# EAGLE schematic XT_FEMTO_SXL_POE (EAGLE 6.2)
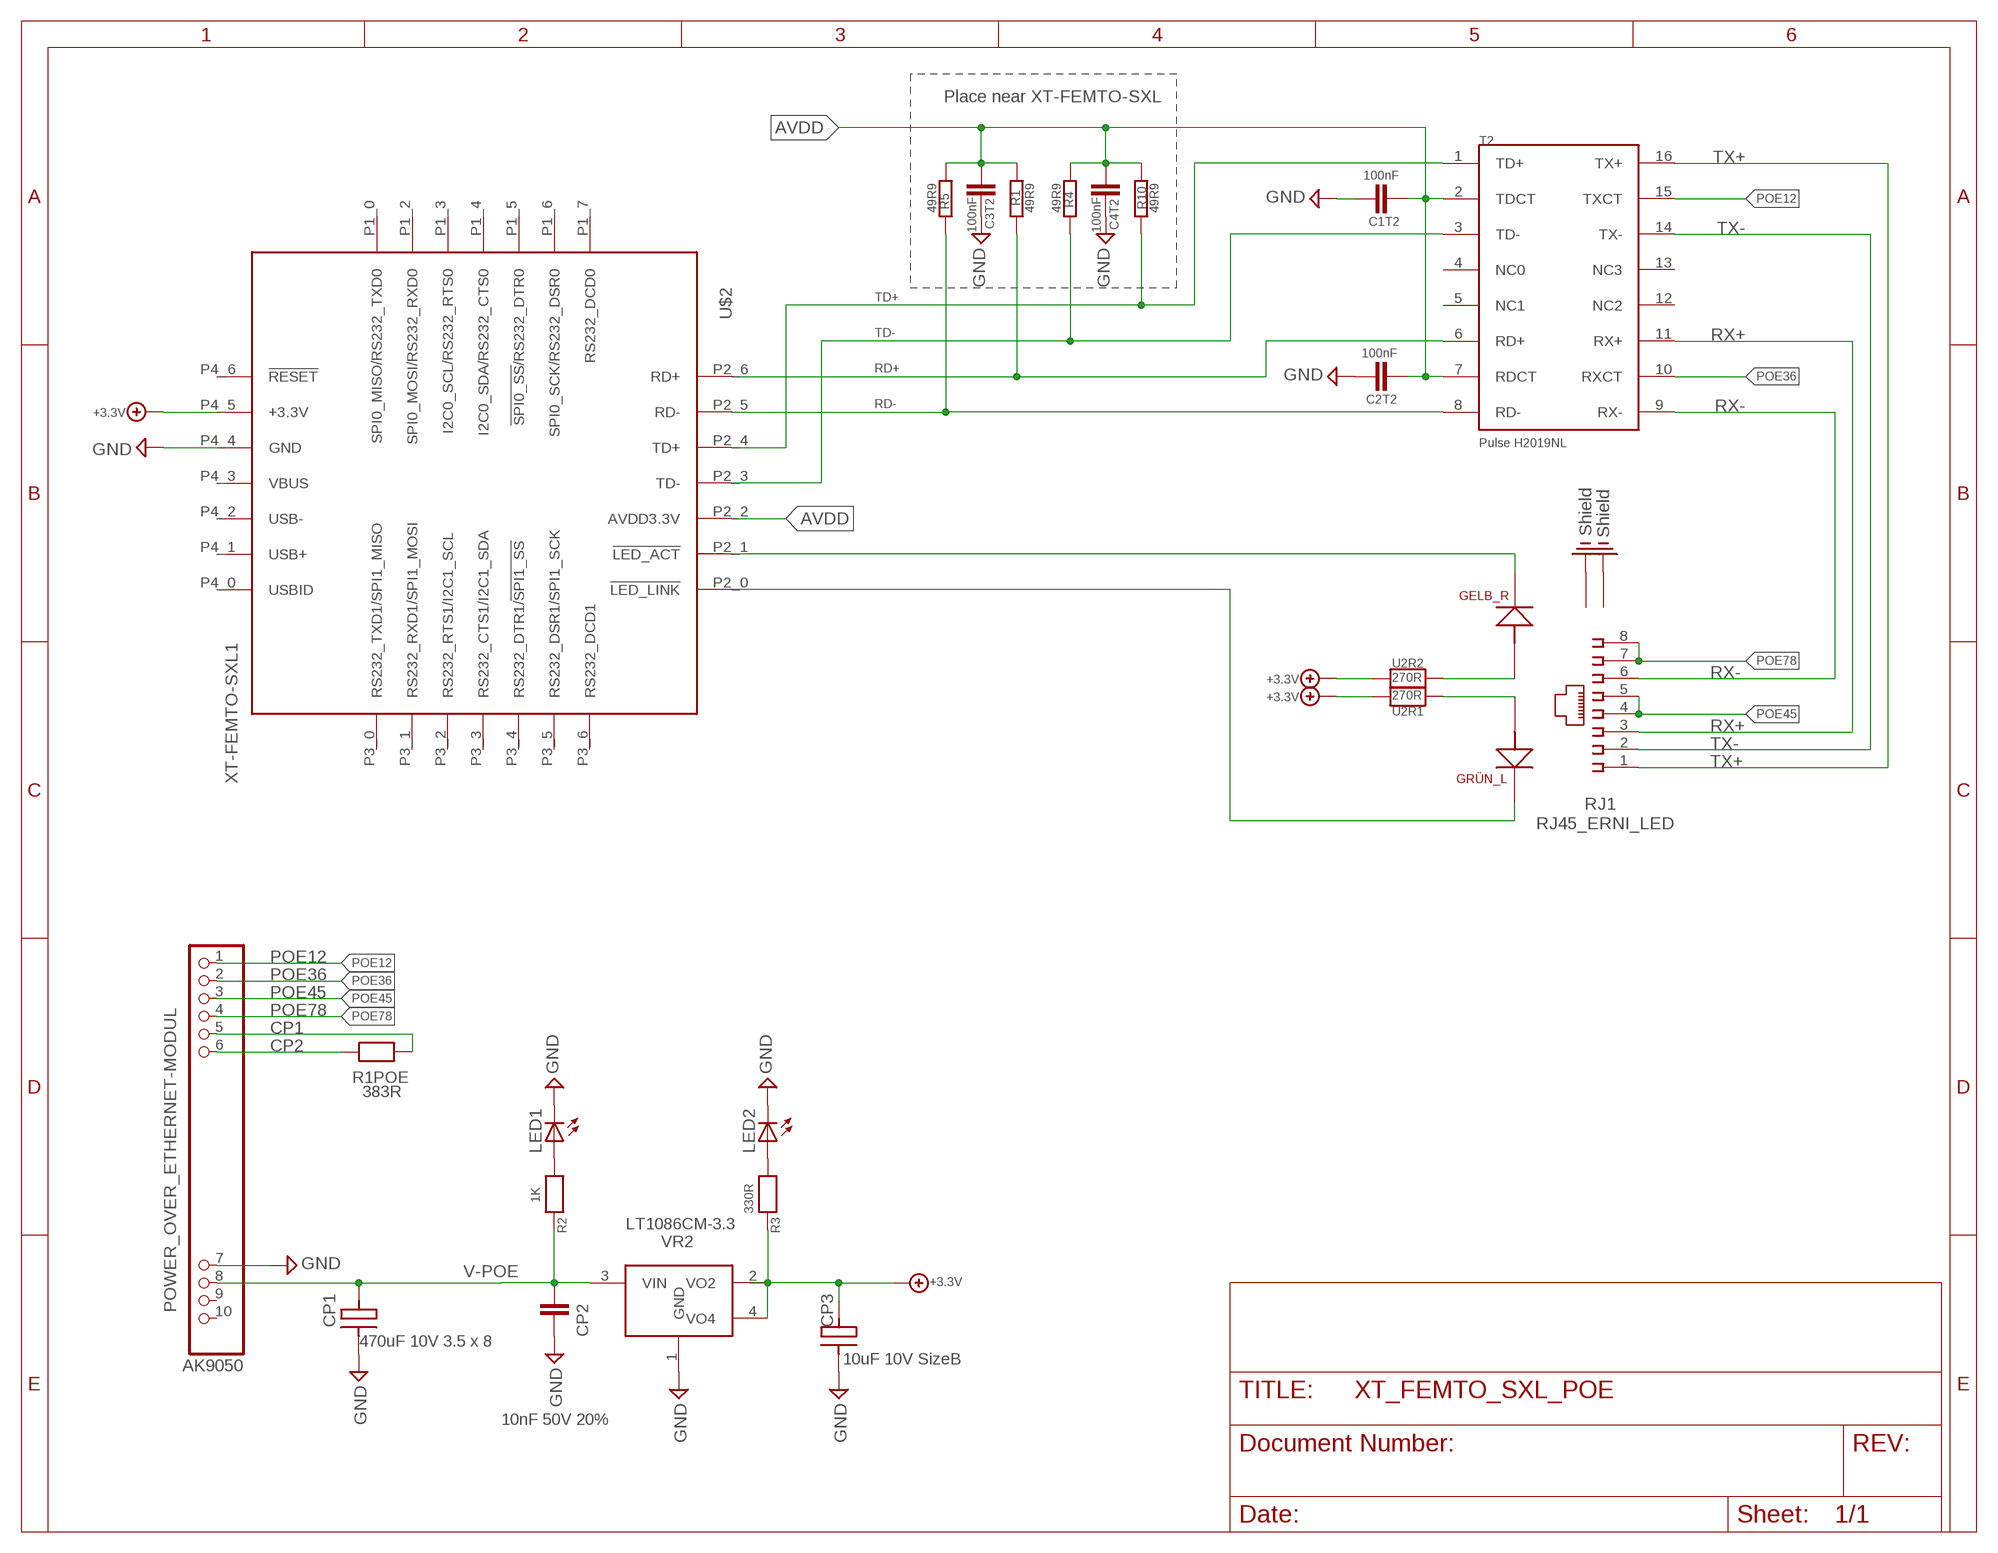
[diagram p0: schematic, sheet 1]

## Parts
C1T2  100nF  CHIP-C-VTS0402  [R0402_VTS]
C2T2  100nF  CHIP-C-VTS0402  [R0402_VTS]
C3T2  100nF  CHIP-C-VTS0402  [R0402_VTS]
C4T2  100nF  CHIP-C-VTS0402  [R0402_VTS]
CP1  470uF 10V 3.5 x 8  C3528_B  [ORCAD_X_CT3528]
CP2  10nF 50V 20%  CHIP-C-0603  [SMD-0603]
CP3  10uF 10V SizeB  C3528_B  [ORCAD_X_CT3528]
LED1  LED3MM  [LED3MM]
LED2  LED3MM  [LED3MM]
POWER_OVER_ETHERNET-MODUL  AK9050  POE_AG9000  [POE_AG9000]
R1  49R9  R-EU_R0603  [R0603]
R1POE  383R  CHIP-R-0603  [SMD-0603]
R2  1K  CHIP-R-0603  [SMD-0603]
R3  330R  CHIP-R-0603  [SMD-0603]
R4  49R9  R-EU_R0603  [R0603]
R5  49R9  R-EU_R0603  [R0603]
R10  49R9  R-EU_R0603  [R0603]
RJ1  RJ45_ERNI_LED  [ORCAD_X_ERNI_RJ45_LED]
T2  Pulse H2019NL  PULSE_H1102  [SOTRANSF]
U2R1  270R  CHIP-R-VTS04020402_VTS  [R0402_VTS]
U2R2  270R  CHIP-R-VTS04020402_VTS  [R0402_VTS]
U$2  XT-FEMTO-SXL1  [XT-FEMTO-SXL-PIN]
VR2  LT1086CM-3.3  LT1086_5.0  [DPAK_223]

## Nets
+3.3V: CP3.1(C+) R3.2 U2R1.2 U2R2.2 U$2.P4_5(+3.3V) VR2.2(VO2) VR2.4(VO4)
AVDD: C1T2.1 C2T2.2 C3T2.1 C4T2.2 R1.2 R4.2 R5.2 R10.2 T2.2(TDCT) T2.7(RDCT) U$2.P2_2(AVDD3.3V)
CP1: POWER_OVER_ETHERNET-MODUL.5(CP1) R1POE.1
CP2: POWER_OVER_ETHERNET-MODUL.6(CP2) R1POE.2
GND: C1T2.2 C2T2.1 C3T2.2 C4T2.1 CP1.2(C-) CP2.1 CP3.2(C-) LED1.K(C) LED2.K(C) POWER_OVER_ETHERNET-MODUL.7(GND) U$2.P4_4(GND) VR2.1(GND)
N$1: CP2.2 R2.2 VR2.3(VIN)
N$2: RJ1.K1 U$2.P2_1(!LED_ACT)
N$5: RJ1.K2 U$2.P2_0(!LED_LINK)
N$6: RJ1.A1 U2R2.1
N$7: RJ1.A2 U2R1.1
N$37: LED1.A R2.1
N$38: LED2.A R3.1
PE: RJ1.9 RJ1.10 ; supply symbol labelled Shield
POE12: POWER_OVER_ETHERNET-MODUL.1(VA1) T2.15(TXCT)
POE36: POWER_OVER_ETHERNET-MODUL.2(VA2) T2.10(RXCT)
POE45: POWER_OVER_ETHERNET-MODUL.3(VB1) RJ1.4 RJ1.5
POE78: POWER_OVER_ETHERNET-MODUL.4(VB2) RJ1.7 RJ1.8
RD+: R1.1 T2.6(RD+) U$2.P2_6(RD+)
RD-: R5.1 T2.8(RD-) U$2.P2_5(RD-)
RX+: RJ1.3 T2.11(RX+)
RX-: RJ1.6 T2.9(RX-)
TD+: R10.1 T2.1(TD+) U$2.P2_4(TD+)
TD-: R4.1 T2.3(TD-) U$2.P2_3(TD-)
TX+: RJ1.1 T2.16(TX+)
TX-: RJ1.2 T2.14(TX-)
V-POE: CP1.1(C+) POWER_OVER_ETHERNET-MODUL.8(VDC+)
Unconnected: POWER_OVER_ETHERNET-MODUL.9(ADJ) POWER_OVER_ETHERNET-MODUL.10(IC) T2.4(NC0) T2.5(NC1) T2.12(NC2) T2.13(NC3) U$2.P1_0(SPI0_MISO/RS232_TXD0) U$2.P1_2(SPI0_MOSI/RS232_RXD0) U$2.P1_3(I2C0_SCL/RS232_RTS0) U$2.P1_4(I2C0_SDA/RS232_CTS0) U$2.P1_5(!SPI0_SS!/RS232_DTR0) U$2.P1_6(SPI0_SCK/RS232_DSR0) U$2.P1_7(RS232_DCD0) U$2.P3_0(RS232_TXD1/SPI1_MISO) U$2.P3_1(RS232_RXD1/SPI1_MOSI) U$2.P3_2(RS232_RTS1/I2C1_SCL) U$2.P3_3(RS232_CTS1/I2C1_SDA) U$2.P3_4(RS232_DTR1/!SPI1_SS!) U$2.P3_5(RS232_DSR1/SPI1_SCK) U$2.P3_6(RS232_DCD1) U$2.P4_0(USBID) U$2.P4_1(USB+) U$2.P4_2(USB-) U$2.P4_3(VBUS) U$2.P4_6(!RESET)

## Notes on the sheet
- Place near XT-FEMTO-SXL
- 10nF 50V 20%

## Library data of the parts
C1T2 C2T2 C3T2 C4T2 CP2 = mea-lib:CHIP-C-?: Chip capacitance
CP1 CP3 = XTMACRO_AS:C3528_B
LED1 LED2 = led:LED: LED
POWER_OVER_ETHERNET-MODUL = XTMACRO:POE_AG9000: PIN HEADER
R1 R4 R5 R10 = rcl:R-EU_: RESISTOR, European symbol
R1POE U2R1 U2R2 = mea-lib:CHIP-R-?: Chip resistors
R2 R3 = XTMACRO:CHIP-R-?: Chip resistors
RJ1 = XTMACRO:RJ45_ERNI_LED
T2 = XTMACRO_AS:PULSE_H1102
U$2 = ak-devices:XT-FEMTO-SXL: AK-NORD XT-FEMTO-SXL
VR2 = XTMACRO_AS:LT1086_5.0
